VAR_GLOBAL
	Nci_Axis                                      : ARRAY[1..AxisNum] OF Axis_Ref; //插补轴
	GroupID				                          : UDINT;    //轴组ID
	ChannelID			                          : UDINT;    //插补通道ID
	NciToPlc	           AT %I*		          : NcToPlc_NciChannel_Ref;
	PlcToNci	           AT %Q*		          : PlcToNc_NciChannel_Ref;
	i                                             : INT;
END_VAR
VAR_GLOBAL CONSTANT
	AxisNum                                       : INT := 3; // 轴数
END_VAR
